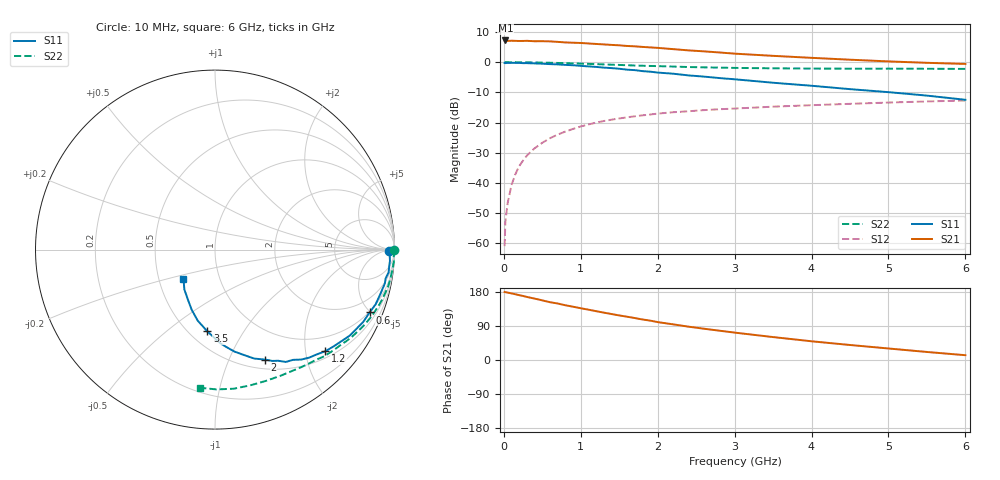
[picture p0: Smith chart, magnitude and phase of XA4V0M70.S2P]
! SIEMENS Discrete & RF Semiconductors
! BFY180
! Si NPN RF Bipolar Junction Transistor in MICRO-X
! VCE = 4 V  IC = 0.7 mA
! Common Emitter S-Parameters:  May  1997
# GHz  S  MA  R  50
!  f  S11  S21  S12  S22
! GHz  MAG  ANG  MAG  ANG  MAG  ANG  MAG  ANG
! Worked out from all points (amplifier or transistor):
!   36 points, 10 MHz to 6 GHz, reference 50 ohm
!   highest |S21| = 7.2 dB at 20 MHz (marker M1)
!   |S21| within 3 dB of that: start of sweep to 2.262 GHz
!   unconditionally stable (mu >= 1): 4.749 GHz to end of sweep
!   at 250 MHz: K = 0.05, MSG = 19.8 dB, |S12| = -32.6 dB
!   at 1.4 GHz: K = 0.43, MSG = 12.4 dB, |S12| = -19.0 dB
!   at 6 GHz: K = 1.04, MAG = 4.9 dB, |S12| = -12.7 dB
!   S11 on the Smith chart (normalised r, x): 10 MHz: 66, -16; 600 MHz: 0.96, -4.94; 1.2 GHz: 0.64, -2.41; 2 GHz: 0.61, -1.37; 3.5 GHz: 0.61, -0.70; 6 GHz: 0.67, -0.23
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0.01  0.972 -0.4  2.27 179.6  0.0009 78.9  0.9975 -0.2
0.02  0.9661 -0.7  2.291 179.0  0.0023 84.2  0.9999 -0.5
0.05  0.9737 -1.7  2.249 177.9  0.0047 85.5  0.9995 -1.2
0.1  0.9767 -3.7  2.268 175.7  0.0093 88.0  0.9954 -2.5
0.15  0.9752 -5.8  2.255 173.5  0.014 86.1  0.9987 -3.7
0.2  0.9755 -7.5  2.245 171.1  0.0191 84.3  0.9964 -4.9
0.3  0.965 -11.2  2.259 166.4  0.0285 82.2  0.9931 -7.3
0.4  0.9547 -14.8  2.223 162.0  0.0376 79.3  0.9904 -9.6
0.6  0.9299 -22.1  2.213 152.5  0.0552 73.6  0.9786 -14.3
1  0.8694 -36.0  2.081 136.6  0.0863 63.0  0.9471 -23.3
1.1  0.8525 -39.3  2.043 132.8  0.0932 60.8  0.9385 -25.2
1.2  0.8354 -42.7  2.005 128.8  0.0999 58.3  0.9291 -27.4
1.5  0.7792 -51.8  1.904 117.6  0.1172 52.1  0.9006 -33.2
2  0.6734 -65.5  1.727 100.0  0.141 43.6  0.8609 -41.7
2.2  0.6453 -70.2  1.646 94.1  0.1483 40.3  0.8474 -44.9
2.4  0.605 -75.2  1.569 88.0  0.1542 37.7  0.8319 -47.8
2.8  0.5467 -83.3  1.45 77.4  0.1664 33.0  0.8136 -53.4
3.5  0.4571 -95.4  1.274 60.5  0.1836 25.9  0.7922 -62.5
4  0.4073 -103.7  1.181 49.4  0.1942 21.2  0.7844 -69.0
4.5  0.3581 -111.4  1.1 39.6  0.2046 17.0  0.7814 -75.6
5.5  0.2799 -127.6  0.977 21.2  0.2239 8.7  0.779 -89.4
6  0.2386 -137.4  0.936 12.7  0.2321 4.3  0.7744 -96.4
